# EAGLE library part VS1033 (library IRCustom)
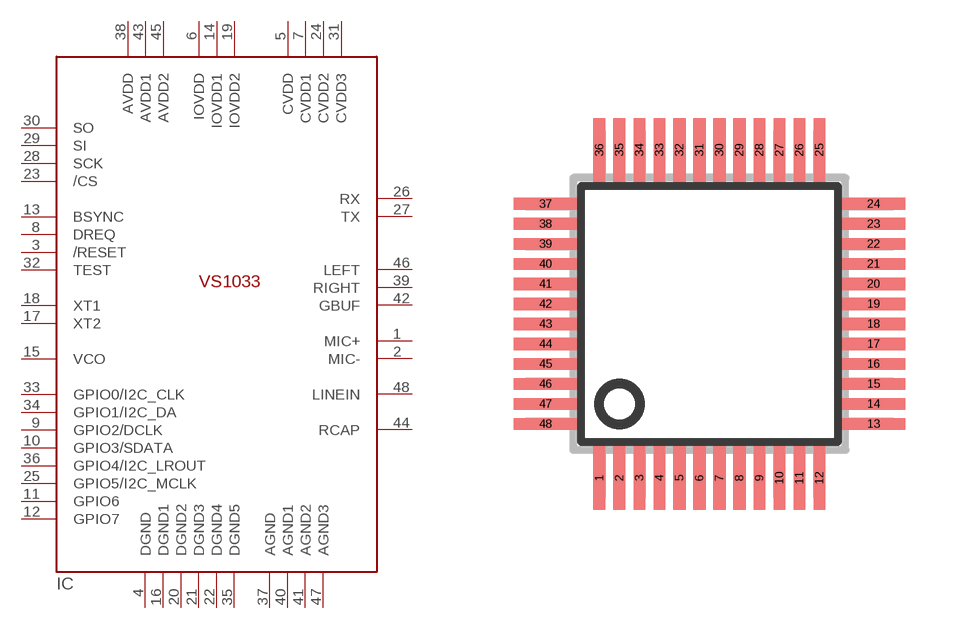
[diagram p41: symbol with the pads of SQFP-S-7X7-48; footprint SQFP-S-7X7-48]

Designator prefix IC

## VS1033  [SQFP-S-7X7-48]
1  MIC+  in
2  MIC-  in
3  /RESET  in
4  DGND  pwr
5  CVDD  pwr
6  IOVDD  pwr
7  CVDD1  pwr
8  DREQ  out
9  GPIO2/DCLK
10  GPIO3/SDATA
11  GPIO6
12  GPIO7
13  BSYNC  in
14  IOVDD1  pwr
15  VCO  out
16  DGND1  pwr
17  XT2  pas
18  XT1  pas
19  IOVDD2  pwr
20  DGND2  pwr
21  DGND3  pwr
22  DGND4  pwr
23  /CS  in
24  CVDD2  pwr
25  GPIO5/I2C_MCLK
26  RX  in
27  TX  out
28  SCK  in
29  SI  in
30  SO  out
31  CVDD3  pwr
32  TEST  in
33  GPIO0/I2C_CLK
34  GPIO1/I2C_DA
35  DGND5  pwr
36  GPIO4/I2C_LROUT
37  AGND  pwr
38  AVDD  pwr
39  RIGHT  out
40  AGND1  pwr
41  AGND2  pwr
42  GBUF  out
43  AVDD1  pwr
44  RCAP  pas
45  AVDD2  pwr
46  LEFT  out
47  AGND3  pwr
48  LINEIN  in

## Footprint SQFP-S-7X7-48 (pad centres in mm)
QFP48 shrink quad flat pack, square
smd 0.3 x 1.6: 1 -2.75,-4.1; 2 -2.25,-4.1; 3 -1.75,-4.1; 4 -1.25,-4.1; 5 -0.75,-4.1; 6 -0.25,-4.1; 7 0.25,-4.1; 8 0.75,-4.1; 9 1.25,-4.1; 10 1.75,-4.1; 11 2.25,-4.1; 12 2.75,-4.1; 25 2.75,4.1; 26 2.25,4.1; 27 1.75,4.1; 28 1.25,4.1; 29 0.75,4.1; 30 0.25,4.1; 31 -0.25,4.1; 32 -0.75,4.1; 33 -1.25,4.1; 34 -1.75,4.1; 35 -2.25,4.1; 36 -2.75,4.1
smd 1.6 x 0.3: 13 4.1,-2.75; 14 4.1,-2.25; 15 4.1,-1.75; 16 4.1,-1.25; 17 4.1,-0.75; 18 4.1,-0.25; 19 4.1,0.25; 20 4.1,0.75; 21 4.1,1.25; 22 4.1,1.75; 23 4.1,2.25; 24 4.1,2.75; 37 -4.1,2.75; 38 -4.1,2.25; 39 -4.1,1.75; 40 -4.1,1.25; 41 -4.1,0.75; 42 -4.1,0.25; 43 -4.1,-0.25; 44 -4.1,-0.75; 45 -4.1,-1.25; 46 -4.1,-1.75; 47 -4.1,-2.25; 48 -4.1,-2.75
